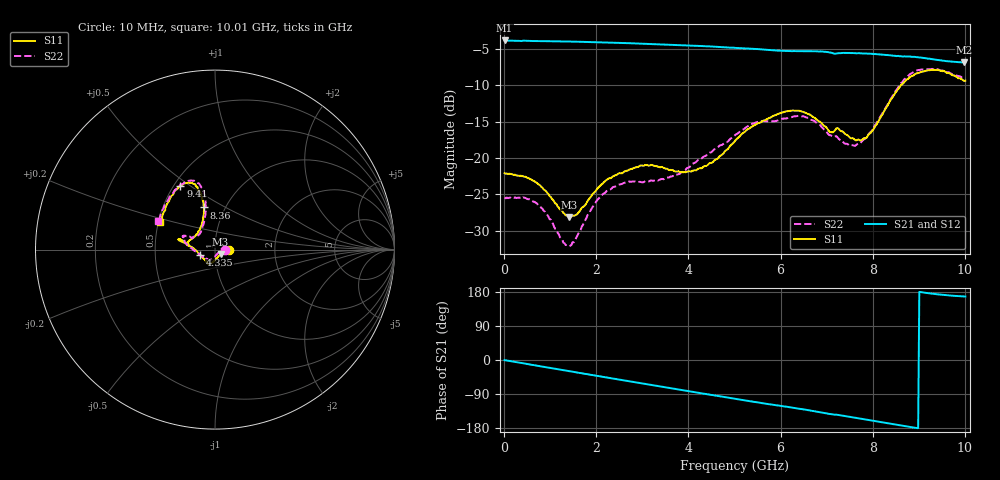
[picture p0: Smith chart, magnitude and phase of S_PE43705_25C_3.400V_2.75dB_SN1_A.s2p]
! Device ID: PE43705
! Serial: 1
! Insertion: A
! Impedance: 50 ohm
! Temp: 25C
! VDD: 3.400V
! Attenuation Step: 2.75dB
#  Hz  S  RI  R  50
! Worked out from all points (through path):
!   401 points, 10 MHz to 10.01 GHz, reference 50 ohm
!   highest |S21| = -3.80 dB at 10 MHz (marker M1); lowest = -6.8 dB at 9.985 GHz (marker M2)
!   group delay of S21, straight-line fit = 54.7 ps
!   lowest |S11| = -28.1 dB at 1.41 GHz (marker M3), VSWR 1.08, Z = 53.2 - j2.54 ohm
!   |S11| at or under -10 dB: start of sweep to 8.605 GHz
!   |S22| runs from -32.1 to -7.7 dB; largest |S21 - S12| = 0.0057
!   S11 on the Smith chart (normalised r, x): 10 MHz: 1.17, -0.00; 4.335 GHz: 0.85, -0.05; 8.36 GHz: 0.80, +0.40; 9.41 GHz: 0.54, +0.46; 10.01 GHz: 0.51, +0.18
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1e7  0.0787 -0.000499  0.646 -0.00331  0.6463 -0.00296  0.0535 -0.000204
6.85e8  0.0673 0.00957  0.6201 -0.1589  0.6201 -0.1584  0.0473 0.0138
1.41e9  0.0313 -0.0239  0.5532 -0.3116  0.5535 -0.3113  0.0187 -0.0161
1.685e9  0.0153 -0.0429  0.5175 -0.3634  0.5176 -0.3634  0.00431 -0.0334
1.985e9  -0.00131 -0.0593  0.4726 -0.4148  0.4727 -0.4148  -0.0118 -0.048
2.26e9  -0.0128 -0.0709  0.4269 -0.4572  0.427 -0.4568  -0.0227 -0.0559
2.96e9  -0.0349 -0.0817  0.2947 -0.5383  0.2952 -0.5381  -0.0433 -0.0532
3.36e9  -0.0413 -0.0765  0.2153 -0.5677  0.2159 -0.5671  -0.0496 -0.0503
3.885e9  -0.0579 -0.055  0.1056 -0.5892  0.1064 -0.5888  -0.0713 -0.0373
4.335e9  -0.0817 -0.0316  0.0114 -0.5902  0.0118 -0.5902  -0.1014 -0.0153
5.01e9  -0.1303 0.0146  -0.1228 -0.5612  -0.1222 -0.5615  -0.1428 0.0161
5.435e9  -0.1646 0.0346  -0.1992 -0.5286  -0.199 -0.5291  -0.1683 0.0449
6.035e9  -0.1972 0.0591  -0.2875 -0.4666  -0.2854 -0.4673  -0.1744 0.0666
6.685e9  -0.1884 0.0446  -0.3794 -0.3901  -0.3793 -0.3897  -0.1653 0.0773
7.085e9  -0.1479 0.0305  -0.4244 -0.3226  -0.4252 -0.3231  -0.1286 0.064
7.61e9  -0.1118 0.0734  -0.4677 -0.2462  -0.4669 -0.2469  -0.0844 0.0871
7.91e9  -0.0826 0.1191  -0.4864 -0.1929  -0.4868 -0.1955  -0.0698 0.1282
8.36e9  -0.0615 0.2351  -0.499 -0.1097  -0.4983 -0.112  -0.0517 0.2419
8.835e9  -0.1028 0.3509  -0.498 -0.0229  -0.4953 -0.0251  -0.0959 0.3707
9.41e9  -0.1928 0.3552  -0.4711 0.0557  -0.47 0.0545  -0.193 0.3611
9.985e9  -0.2967 0.1656  -0.445 0.097  -0.4465 0.0977  -0.3094 0.1704
1.001e10  -0.3041 0.155  -0.4459 0.099  -0.4479 0.0982  -0.317 0.1578
